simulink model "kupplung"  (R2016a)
settings: Solver=ode45  StartTime=0.0  StopTime=15  FixedStep=1e-4  RelTol=1e-3
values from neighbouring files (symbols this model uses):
  M = block.DialogPrm(1).Data    [sfun_inferenz.m]
undefined symbols (not defined in the file or in its folder): J, Mg, Mh, w0, wl0, wr0
libraries: simulink x1

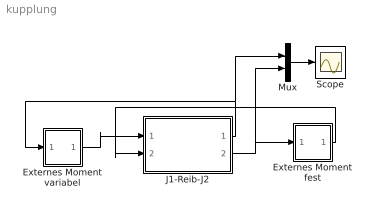
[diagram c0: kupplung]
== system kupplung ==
  Externes Moment fest : Subsystem
  Externes Moment variabel : Subsystem
  J1-Reib-J2 : Subsystem
  Mux : Mux  Inputs=2
  Scope : Scope
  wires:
  Externes Moment variabel/1(M) -> J1-Reib-J2/1(Ml)
  J1-Reib-J2/2(wr) -> Externes Moment fest/1(w), Mux/2
  J1-Reib-J2/1(wl) -> Externes Moment variabel/1(w), Mux/1
  Externes Moment fest/1(M) -> J1-Reib-J2/2(Mr)
  Mux/1 -> Scope/1

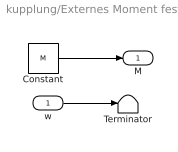
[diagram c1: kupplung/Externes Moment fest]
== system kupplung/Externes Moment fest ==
  w : Inport
  Constant : Constant  Value=M
  Terminator : Terminator
  M : Outport
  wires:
  Constant/1 -> M/1
  w/1 -> Terminator/1

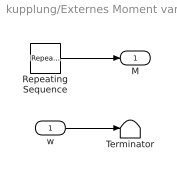
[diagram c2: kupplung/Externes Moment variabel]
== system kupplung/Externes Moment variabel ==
  w : Inport
  Repeating Sequence : simulink/Sources/Repeating Sequence  SystemSampleTime=-1  rep_seq_t=tvek  rep_seq_y=Mvek
  Terminator : Terminator
  M : Outport
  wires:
  Repeating Sequence/1 -> M/1
  w/1 -> Terminator/1

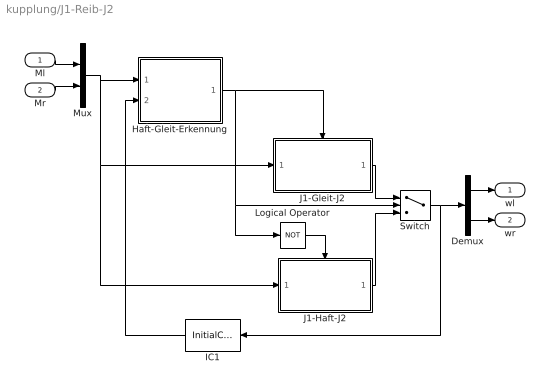
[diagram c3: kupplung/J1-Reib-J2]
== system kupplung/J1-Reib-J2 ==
  note: .
  Ml : Inport
  Mr : Inport  Port=2
  Demux : Demux  Outputs=2
  Haft-Gleit-Erkennung : Subsystem
  IC1 : InitialCondition  Value=[wl0 wr0]
  J1-Gleit-J2 : Subsystem
  J1-Haft-J2 : Subsystem
  Logical Operator : Logic  Operator=NOT  AllPortsSameDT=off
  Mux : Mux  Inputs=2
  Switch : Switch  Threshold=0.5
  wl : Outport
  wr : Outport  Port=2
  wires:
  Haft-Gleit-Erkennung/1(gleitet) -> Switch/2, Logical Operator/1, J1-Gleit-J2/Enable
  J1-Haft-J2/1(w) -> Switch/3
  Switch/1 -> Demux/1, IC1/1
  Logical Operator/1 -> J1-Haft-J2/Enable
  Ml/1 -> Mux/1
  Mr/1 -> Mux/2
  Mux/1 -> Haft-Gleit-Erkennung/1(M), J1-Haft-J2/1(M), J1-Gleit-J2/1(M)
  Demux/1 -> wl/1
  Demux/2 -> wr/1
  J1-Gleit-J2/1(w) -> Switch/1
  IC1/1 -> Haft-Gleit-Erkennung/2(w)

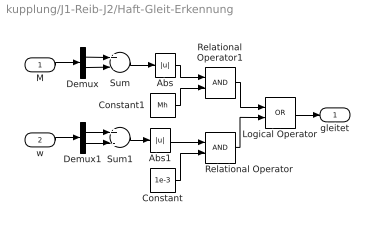
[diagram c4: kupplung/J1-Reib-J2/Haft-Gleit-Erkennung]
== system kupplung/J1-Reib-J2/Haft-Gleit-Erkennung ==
  note: .
  M : Inport
  w : Inport  Port=2
  Abs : Abs
  Abs1 : Abs
  Constant : Constant  Value=1e-3
  Constant1 : Constant  Value=Mh
  Demux : Demux  Outputs=2
  Demux1 : Demux  Outputs=2
  Logical Operator : Logic  Operator=OR  AllPortsSameDT=off
  Relational Operator : RelationalOperator
  Relational Operator1 : RelationalOperator
  Sum : Sum  Inputs=+-
  Sum1 : Sum  Inputs=+-
  gleitet : Outport
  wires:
  Logical Operator/1 -> gleitet/1
  Sum/1 -> Abs/1
  Sum1/1 -> Abs1/1
  Constant/1 -> Relational Operator/2
  Abs1/1 -> Relational Operator/1
  Abs/1 -> Relational Operator1/1
  Constant1/1 -> Relational Operator1/2
  Relational Operator1/1 -> Logical Operator/1
  Relational Operator/1 -> Logical Operator/2
  M/1 -> Demux/1
  Demux/1 -> Sum/1
  Demux/2 -> Sum/2
  Demux1/1 -> Sum1/1
  Demux1/2 -> Sum1/2
  w/1 -> Demux1/1

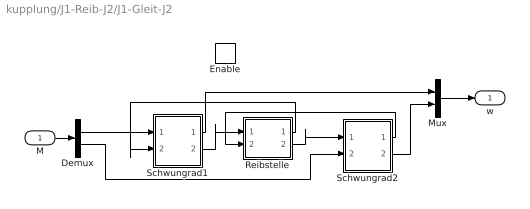
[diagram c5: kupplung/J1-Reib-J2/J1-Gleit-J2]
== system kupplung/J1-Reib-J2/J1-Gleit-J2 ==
  note: .
  M : Inport
  Enable : EnablePort  StatesWhenEnabling=reset
  Demux : Demux  Outputs=2
  Mux : Mux  Inputs=2
  Reibstelle : Subsystem
  Schwungrad1 : Subsystem
  Schwungrad2 : Subsystem
  w : Outport
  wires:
  Schwungrad2/1(wl) -> Reibstelle/2(wr)
  Reibstelle/2(Mr) -> Schwungrad2/1(Ml)
  M/1 -> Demux/1
  Demux/2 -> Schwungrad2/2(Mr)
  Mux/1 -> w/1
  Schwungrad2/2(wr) -> Mux/2
  Schwungrad1/1(wl) -> Mux/1
  Schwungrad1/2(wr) -> Reibstelle/1(wl)
  Reibstelle/1(Ml) -> Schwungrad1/2(Mr)
  Demux/1 -> Schwungrad1/1(Ml)

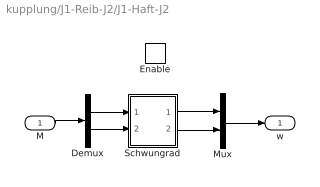
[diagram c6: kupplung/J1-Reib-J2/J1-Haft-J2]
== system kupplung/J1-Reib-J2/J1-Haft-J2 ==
  note: .
  M : Inport
  Enable : EnablePort  StatesWhenEnabling=reset
  Demux : Demux  Outputs=2
  Mux : Mux  Inputs=2
  Schwungrad : Subsystem
  w : Outport
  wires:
  M/1 -> Demux/1
  Demux/1 -> Schwungrad/1(Ml)
  Schwungrad/1(wl) -> Mux/1
  Schwungrad/2(wr) -> Mux/2
  Mux/1 -> w/1
  Demux/2 -> Schwungrad/2(Mr)

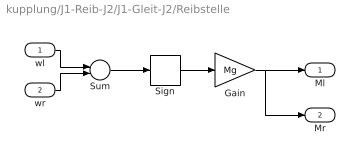
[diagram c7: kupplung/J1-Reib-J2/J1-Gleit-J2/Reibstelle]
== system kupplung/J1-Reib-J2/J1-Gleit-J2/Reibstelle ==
  wl : Inport
  wr : Inport  Port=2
  Gain : Gain  Gain=Mg
  Sign : Signum
  Sum : Sum  Inputs=+-
  Ml : Outport
  Mr : Outport  Port=2
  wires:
  Gain/1 -> Mr/1, Ml/1
  Sign/1 -> Gain/1
  Sum/1 -> Sign/1
  wl/1 -> Sum/1
  wr/1 -> Sum/2

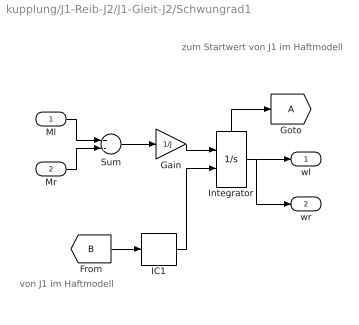
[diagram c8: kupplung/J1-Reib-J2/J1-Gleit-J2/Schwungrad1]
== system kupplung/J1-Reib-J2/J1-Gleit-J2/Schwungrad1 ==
  note: zum Startwert von J1 im Haftmodell
  note: von J1 im Haftmodell
  note: .
  Ml : Inport
  Mr : Inport  Port=2
  Gain : Gain  Gain=1/J
  Goto : Goto  TagVisibility=global
  IC1 : InitialCondition  Value=wl0
  Integrator : Integrator  InitialConditionSource=external  InitialCondition=w0  ShowStatePort=on
  Sum : Sum  Inputs=+-
  wl : Outport
  wr : Outport  Port=2
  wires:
  Integrator/1 -> wl/1, wr/1
  Gain/1 -> Integrator/1
  Sum/1 -> Gain/1
  Mr/1 -> Sum/2
  Ml/1 -> Sum/1
  Integrator/State -> Goto/1
  [B] -> IC1/1
  IC1/1 -> Integrator/2

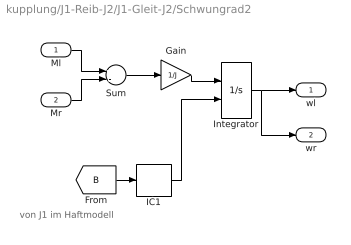
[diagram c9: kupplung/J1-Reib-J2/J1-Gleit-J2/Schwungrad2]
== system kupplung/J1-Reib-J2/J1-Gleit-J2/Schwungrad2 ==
  note: von J1 im Haftmodell
  Ml : Inport
  Mr : Inport  Port=2
  Gain : Gain  Gain=1/J
  IC1 : InitialCondition  Value=wr0
  Integrator : Integrator  InitialConditionSource=external  InitialCondition=w0
  Sum : Sum  Inputs=+-
  wl : Outport
  wr : Outport  Port=2
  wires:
  Ml/1 -> Sum/1
  Mr/1 -> Sum/2
  Sum/1 -> Gain/1
  Gain/1 -> Integrator/1
  Integrator/1 -> wr/1, wl/1
  [B] -> IC1/1
  IC1/1 -> Integrator/2

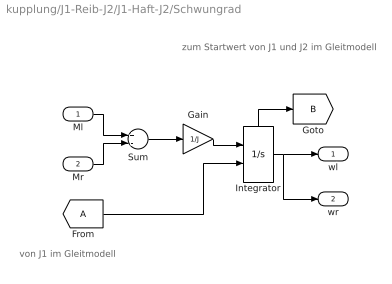
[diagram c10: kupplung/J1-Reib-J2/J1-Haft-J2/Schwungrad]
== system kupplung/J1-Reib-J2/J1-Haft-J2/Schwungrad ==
  note: von J1 im Gleitmodell
  note: zum Startwert von J1 und J2 im Gleitmodell
  Ml : Inport
  Mr : Inport  Port=2
  From : From  TagVisibility=global
  Gain : Gain  Gain=1/J
  Integrator : Integrator  InitialConditionSource=external  InitialCondition=w0  ShowStatePort=on
  Sum : Sum  Inputs=+-
  wl : Outport
  wr : Outport  Port=2
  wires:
  Integrator/1 -> wl/1, wr/1
  Gain/1 -> Integrator/1
  Sum/1 -> Gain/1
  Mr/1 -> Sum/2
  Ml/1 -> Sum/1
  From/1 -> Integrator/2
  Integrator/State -> [B]
